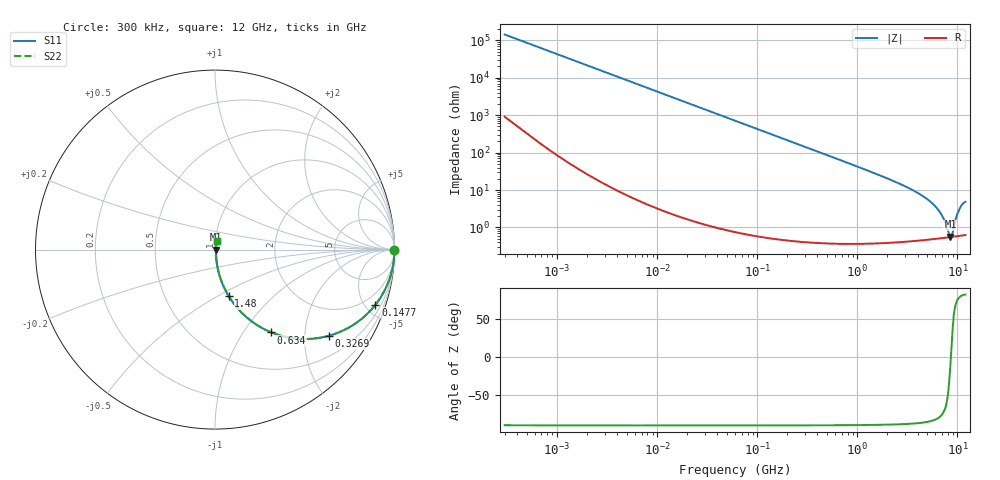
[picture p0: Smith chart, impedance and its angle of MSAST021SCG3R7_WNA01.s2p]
! MSAST021SCG3R7_WNA01  S-PARAMETER MODEL  ( General Type )
! Model Generated by TAIYO YUDEN Corporation (http://www.ty-top.com)
! Version 2.0
! TAIYO YUDEN Control No. 181101
! Copyright(c) 2015 TAIYO YUDEN CO.,LTD. All Rights Reserved.
! Product Description (link to TY-COMPAS)
! https://ds.yuden.co.jp/TYCOMPAS/or/detail?pn=MSAST021SCG3R7BWNA01&u=M
! Products Name : Multilayer Ceramic Capacitors
! Characteristics :
!  Capacitance : 3.7 pF , Rated Voltage : 25V , TCC : CG / C0G
!  Case Size : 0.25 x 0.125 / 0.0098 x 0.0049 [mm/inch] , Thickness : 0.125 / 0.0049 [mm/inch]
!  (Conditions: Temperature = 25 degC , DC Bias Current/Voltage = 0A / 0V)
! External Node Assignments :
!  1  o---| |---o  2
! GND o---------o GND
! Frequency Range : 0.3MHz  -  12000MHz  [ 401 STEP ]
# MHz S RI R 50
! Freq[MHz].  S11 Real  S11 Imag  S21 Real  S21 Imag  S12 Real  S12 Imag  S22 Real  S22 Imag
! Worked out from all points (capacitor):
!   401 points, 300 kHz to 12 GHz, reference 50 ohm
!   read as one part in series: C = 3.7 pF near 316.3 kHz
!   lowest |Z| = 563 mohm at 8.504 GHz (marker M1)
!   series resonance near 8.598 GHz, so ESL is about 93 pH
!   S11 on the Smith chart (normalised r, x): 300 kHz: open; 147.7 MHz: 1.01, -5.82; 326.9 MHz: 1.01, -2.63; 634 MHz: 1.01, -1.35; 1.48 GHz: 1.01, -0.56; 12 GHz: 1.01, +0.10
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0.3  1 -0.000697  4.91e-06 0.000697  4.91e-06 0.000697  1 -0.000697
1.769972  1 -0.00411  2.24e-05 0.00411  2.24e-05 0.00411  1 -0.00411
10.44266  0.9994 -0.0243  0.000607 0.0243  0.000607 0.0243  0.9994 -0.0243
60  0.9808 -0.1368  0.0192 0.1368  0.0192 0.1368  0.9808 -0.1368
147.6816  0.8941 -0.3069  0.1059 0.3069  0.1059 0.3069  0.8941 -0.3069
326.9496  0.6328 -0.4805  0.3672 0.4805  0.3672 0.4805  0.6328 -0.4805
353.9943  0.5951 -0.4893  0.4049 0.4893  0.4049 0.4893  0.5951 -0.4893
634.0297  0.3138 -0.4613  0.6862 0.4613  0.6862 0.4613  0.3138 -0.4613
968.706  0.1632 -0.3655  0.8368 0.3655  0.8368 0.3655  0.1632 -0.3655
1480.043  0.0766 -0.2594  0.9234 0.2594  0.9234 0.2594  0.0766 -0.2594
2088.533  0.0396 -0.1853  0.9604 0.1853  0.9604 0.1853  0.0396 -0.1853
3841.137  0.0122 -0.088  0.9878 0.088  0.9878 0.088  0.0122 -0.088
5565.855  0.00677 -0.0441  0.9932 0.0441  0.9932 0.0441  0.00677 -0.0441
6879.757  0.00561 -0.0219  0.9944 0.0219  0.9944 0.0219  0.00561 -0.0219
7448.838  0.00546 -0.0139  0.9945 0.0139  0.9945 0.0139  0.00546 -0.0139
8281.503  0.00547 -0.00328  0.9945 0.00328  0.9945 0.00328  0.00547 -0.00328
8503.825  0.00551 -0.00102  0.9945 0.00102  0.9945 0.00102  0.00551 -0.00102
8966.534  0.00563 0.00446  0.9944 -0.00446  0.9944 -0.00446  0.00563 0.00446
9708.23  0.00608 0.0173  0.9939 -0.0173  0.9939 -0.0173  0.00608 0.0173
10511.28  0.00689 0.0306  0.9931 -0.0306  0.9931 -0.0306  0.00689 0.0306
11380.75  0.00796 0.0427  0.992 -0.0427  0.992 -0.0427  0.00796 0.0427
12000  0.00848 0.0471  0.9915 -0.0471  0.9915 -0.0471  0.00848 0.0471
